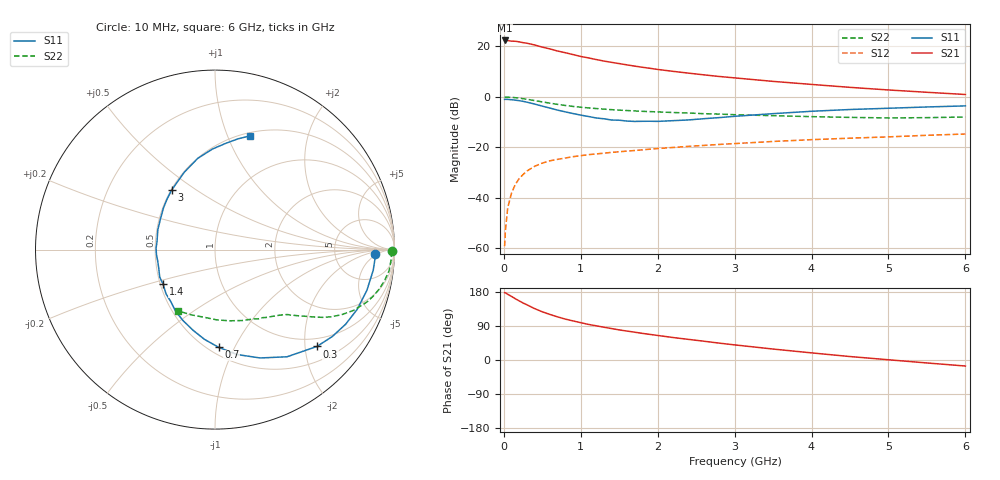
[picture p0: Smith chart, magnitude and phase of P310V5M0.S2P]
! SIEMENS Small Signal Semiconductors
! BFP181
! Si NPN RF Bipolar Junction Transistor in SOT143
! VCE = 10 V  IC = 5 mA
! Common Emitter S-Parameters:  March  1996
# GHz  S  MA  R  50
!  f  S11  S21  S12  S22
! GHz  MAG  ANG  MAG  ANG  MAG  ANG  MAG  ANG
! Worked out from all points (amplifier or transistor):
!   36 points, 10 MHz to 6 GHz, reference 50 ohm
!   highest |S21| = 22.3 dB at 10 MHz (marker M1)
!   |S21| within 3 dB of that: start of sweep to 550.4 MHz
!   unconditionally stable (mu >= 1): 1.902 GHz to end of sweep
!   at 250 MHz: K = 0.21, MSG = 26.1 dB, |S12| = -30.8 dB
!   at 1.4 GHz: K = 0.86, MSG = 17.8 dB, |S12| = -22.0 dB
!   at 6 GHz: K = 1.08, MAG = 6.1 dB, |S12| = -14.7 dB
!   S11 on the Smith chart (normalised r, x): 10 MHz: 16, -4; 300 MHz: 0.81, -2.26; 700 MHz: 0.56, -0.87; 1.4 GHz: 0.52, -0.23; 3 GHz: 0.50, +0.40; 6 GHz: 0.53, +1.20
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0.01  0.8891 -1.5  13.08 177.8  0.0011 71.5  0.9869 -0.6
0.02  0.8932 -3.0  13.07 177.3  0.0022 87.0  0.9847 -1.3
0.05  0.8891 -7.4  13.02 173.5  0.0063 89.0  0.9825 -3.5
0.1  0.8762 -15.0  12.67 167.8  0.0124 79.3  0.9771 -7.0
0.15  0.8594 -22.8  12.6 161.6  0.0185 77.6  0.9603 -10.4
0.2  0.8383 -29.7  12.26 155.9  0.0241 73.1  0.9412 -13.5
0.3  0.7836 -43.5  11.54 145.7  0.0339 66.0  0.8947 -19.1
0.4  0.7195 -56.1  10.64 135.6  0.042 60.6  0.8427 -23.7
0.5  0.654 -67.4  9.651 127.2  0.0487 55.6  0.7934 -27.2
0.6  0.5975 -78.1  8.891 120.1  0.054 52.4  0.7486 -30.0
0.7  0.5447 -87.9  8.065 113.7  0.0578 49.6  0.7083 -32.2
0.8  0.5034 -96.7  7.47 107.9  0.0614 47.2  0.674 -33.9
0.9  0.4663 -105.1  6.863 103.1  0.0652 45.2  0.645 -35.4
1.1  0.4077 -122.6  5.904 93.9  0.0715 42.7  0.6029 -37.8
1.4  0.3473 -146.3  4.819 83.0  0.0794 40.2  0.557 -40.9
1.8  0.3274 -175.5  3.855 70.3  0.089 38.4  0.5166 -44.9
2.2  0.3371 160.9  3.196 59.3  0.0992 36.5  0.489 -49.6
3  0.4109 125.9  2.372 39.9  0.1185 32.1  0.4424 -60.7
3.5  0.464 111.6  2.022 28.9  0.1305 29.2  0.423 -69.1
4.5  0.5607 91.4  1.54 9.1  0.1516 22.2  0.3913 -88.9
5.5  0.6296 78.4  1.23 -7.8  0.1729 16.6  0.3868 -110.0
6  0.6614 73.1  1.112 -15.9  0.1834 12.9  0.3982 -121.0
